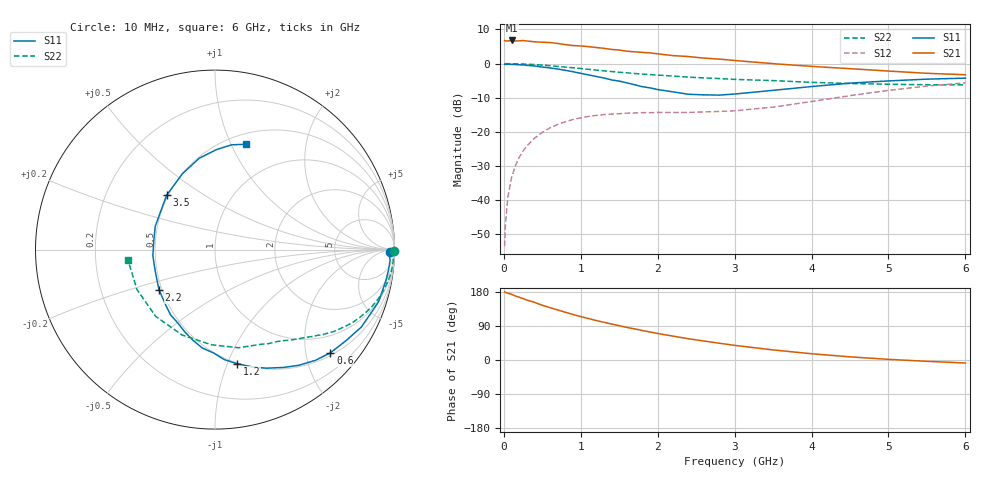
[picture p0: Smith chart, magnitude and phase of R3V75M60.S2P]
! SIEMENS Small Signal Semiconductors
! BFR181
! Si NPN RF Bipolar Junction Transistor in SOT23
! VCE = 0.75 V  IC = 0.6 mA
! Common Emitter S-Parameters:  May  1996
# GHz  S  MA  R  50
!  f  S11  S21  S12  S22
! GHz  MAG  ANG  MAG  ANG  MAG  ANG  MAG  ANG
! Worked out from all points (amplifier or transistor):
!   36 points, 10 MHz to 6 GHz, reference 50 ohm
!   highest |S21| = 6.8 dB at 100 MHz (marker M1)
!   |S21| within 3 dB of that: start of sweep to 1.553 GHz
!   unconditionally stable (mu >= 1): 2.168 GHz to 4.286 GHz
!   at 250 MHz: K = 0.13, MSG = 16.2 dB, |S12| = -25.6 dB
!   at 1.4 GHz: K = 0.68, MSG = 9.5 dB, |S12| = -14.8 dB
!   at 6 GHz: K = 0.97, MSG = 1.2 dB, |S12| = -5.7 dB
!   S11 on the Smith chart (normalised r, x): 10 MHz: 60, -33; 600 MHz: 0.56, -2.51; 1.2 GHz: 0.50, -1.08; 2.2 GHz: 0.48, -0.26; 3.5 GHz: 0.49, +0.36; 6 GHz: 0.61, +1.14
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0.01  0.9749 -0.8  2.178 179.7  0.0021 97.8  0.9986 -0.4
0.02  0.9724 -1.4  2.146 178.4  0.0042 87.5  0.9943 -0.7
0.05  0.9774 -3.6  2.146 176.6  0.0107 86.2  0.9968 -1.7
0.1  0.9732 -6.9  2.183 173.3  0.0212 85.5  0.9951 -3.5
0.15  0.9673 -10.6  2.142 168.9  0.0318 82.4  0.9926 -5.4
0.25  0.9566 -17.6  2.179 161.9  0.0524 78.0  0.9854 -8.8
0.4  0.9224 -27.9  2.084 152.1  0.0807 71.0  0.9666 -13.7
0.5  0.8889 -34.8  2.055 144.4  0.0982 66.3  0.9492 -16.9
0.6  0.8625 -41.8  2.034 138.1  0.1143 62.1  0.9293 -20.1
0.8  0.7958 -54.1  1.897 126.0  0.1404 54.4  0.8877 -25.5
1.1  0.6831 -72.8  1.772 109.4  0.1678 45.0  0.8241 -32.4
1.2  0.6476 -79.0  1.72 104.2  0.1735 42.1  0.8031 -34.7
1.5  0.5532 -97.2  1.58 90.6  0.1838 36.2  0.7445 -39.9
1.6  0.5208 -103.5  1.516 85.9  0.1874 34.7  0.7322 -41.3
1.9  0.4405 -124.0  1.433 73.9  0.1903 32.0  0.6882 -45.9
2.2  0.3848 -144.0  1.308 63.0  0.1919 30.8  0.6553 -50.4
2.4  0.3548 -159.6  1.268 56.1  0.192 31.6  0.6324 -53.4
2.8  0.345 170.7  1.163 44.3  0.1984 34.2  0.6031 -60.3
3.5  0.4053 131.7  0.997 26.6  0.2298 40.5  0.5626 -76.4
4.5  0.5166 99.8  0.842 8.3  0.3389 41.5  0.5099 -111.1
5.5  0.5912 81.0  0.72 -3.5  0.4677 29.9  0.4884 -152.8
6  0.6115 73.6  0.686 -7.9  0.5217 21.9  0.4888 -173.4
